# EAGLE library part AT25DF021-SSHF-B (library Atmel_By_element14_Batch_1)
Two-wire Serial EEPROM
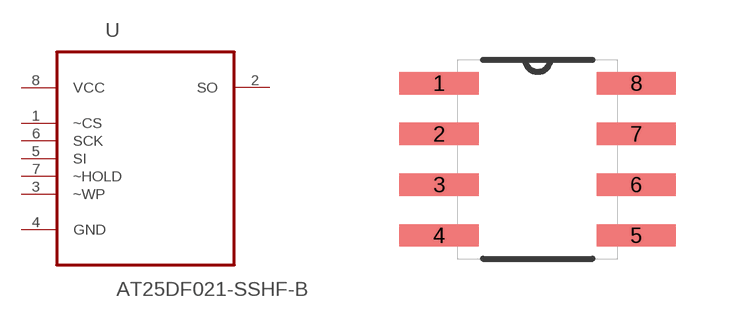
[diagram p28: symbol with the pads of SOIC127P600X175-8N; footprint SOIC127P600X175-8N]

Designator prefix U

## AT25DF021-SSHF-B (MPN: AT25DF021-SSHF-B; OC_FARNELL: 1715439; OC_NEWARK: 15R0304; PACKAGE: SOIC-8; SUPPLIER: Atmel)  [SOIC127P600X175-8N]
1  ~CS  in
2  SO  out
3  ~WP  in
4  GND  pas
5  SI  in
6  SCK  in
7  ~HOLD  in
8  VCC  pwr

## Footprint SOIC127P600X175-8N (pad centres in mm)
smd 1.981 x 0.559: 1 -2.464,1.905; 2 -2.464,0.635; 3 -2.464,-0.635; 4 -2.464,-1.905; 5 2.464,-1.905; 6 2.464,-0.635; 7 2.464,0.635; 8 2.464,1.905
